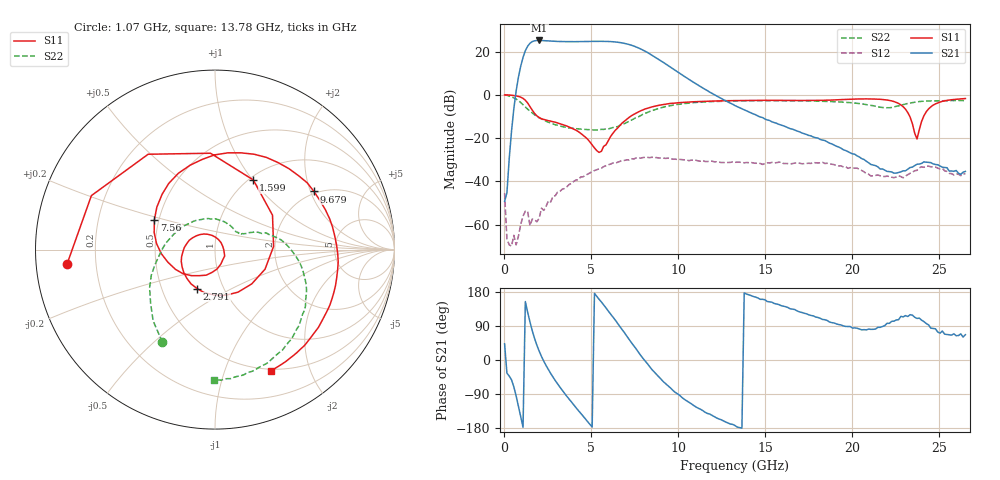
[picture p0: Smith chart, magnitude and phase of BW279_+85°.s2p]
!Agilent Technologies,N5242A,MY52422126,A.09.90.01
!Agilent N5242A: A.09.90.01
!Date: Wednesday, January 15, 2014 09:09:21
!Correction: S11(Full 2 Port with power(1,2))
!S21(Full 2 Port with power(1,2))
!S12(Full 2 Port with power(1,2))
!S22(Full 2 Port with power(1,2))
!S2P File: Measurements: S11, S21, S12, S22:
# Hz S  dB  R 50
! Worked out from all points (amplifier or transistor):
!   201 points, 10 MHz to 26.5 GHz, reference 50 ohm
!   highest |S21| = 25.2 dB at 1.997 GHz (marker M1)
!   |S21| within 3 dB of that: 1.313 GHz to 7.571 GHz (6.259 GHz wide, 141 % of centre)
!   unconditionally stable (mu >= 1): start of sweep to end of sweep
!   at 4.381 GHz: K = 2.34, MAG = 24.8 dB, |S12| = -38.0 dB
!   at 13.26 GHz: K = 7.43, MAG = 1.4 dB, |S12| = -31.2 dB
!   at 26.5 GHz: K = 297.82, MAG = -27.2 dB, |S12| = -36.6 dB
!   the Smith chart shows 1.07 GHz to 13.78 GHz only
!   S11 on the Smith chart (normalised r, x): 1.07 GHz: 0.09, -0.05; 1.599 GHz: 1.04, +1.01; 2.791 GHz: 0.75, -0.35; 7.56 GHz: 0.47, +0.18; 9.679 GHz: 1.93, +2.12; 13.78 GHz: 0.48, -1.45
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1e7  -0.02 -1.3  -49.25 42.8  -45.53 144.0  -0.00 -1.1
6.7225e8  -0.49 -100.9  1.75 -94.7  -69.36 86.6  -1.93 -79.1
1.0696e9  -1.63 -174.3  17.33 -177.4  -56.06 146.8  -4.54 -119.6
1.3345e9  -3.76 125.0  22.50 126.0  -53.85 92.3  -6.60 -140.1
1.5994e9  -7.07 61.3  24.63 77.3  -57.46 100.9  -8.35 -158.2
1.99675e9  -10.47 -21.4  25.16 23.5  -57.08 117.4  -10.61 179.8
2.3941e9  -11.66 -77.2  25.00 -14.7  -51.57 131.6  -12.18 159.9
2.79145e9  -12.44 -114.8  24.81 -45.3  -46.89 134.1  -13.40 140.2
3.58615e9  -14.41 -168.0  24.61 -95.8  -42.53 114.3  -15.04 102.1
4.5133e9  -18.61 134.1  24.65 -147.6  -37.92 88.1  -15.97 64.0
5.308e9  -25.78 49.3  24.74 167.9  -34.63 69.8  -16.29 41.7
6.23515e9  -17.77 -98.1  24.57 113.6  -31.51 42.3  -15.12 30.6
6.8974e9  -12.17 -153.5  23.82 72.2  -30.32 22.0  -13.32 26.0
7.55965e9  -8.49 153.7  22.20 30.0  -29.20 2.0  -10.48 18.3
8.2219e9  -6.19 106.4  19.61 -9.8  -28.91 -17.9  -8.14 5.2
8.88415e9  -4.82 67.7  16.29 -44.7  -29.20 -37.6  -6.24 -10.5
9.67885e9  -3.88 30.4  12.07 -79.8  -29.70 -54.8  -4.78 -28.8
1.3255e10  -2.64 -57.6  -4.97 -173.0  -31.17 -111.9  -2.83 -84.8
1.37848e10  -2.58 -65.3  -6.95 176.9  -31.41 -117.9  -2.77 -90.3
1.77583e10  -2.57 -103.8  -19.51 116.4  -31.21 -175.0  -2.85 -122.7
2.212915e10  -2.56 -150.5  -35.48 96.7  -37.73 132.3  -5.95 -131.3
2.65e10  -1.70 -123.7  -35.40 66.8  -36.55 75.0  -2.72 -149.4
